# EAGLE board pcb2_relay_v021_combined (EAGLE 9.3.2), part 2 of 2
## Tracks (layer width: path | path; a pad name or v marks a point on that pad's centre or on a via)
+5V  (via drill 0.35)
  Top 0.508: IC1.16 20.95,33.66 21.59,34.29 v21.59,34.81
  Top 0.61: 17.78,26.04 v17.78,15.24 17.78,7.49 18.29,6.99 IC3.10 | 17.78,26.04 17.78,26.85 16.87,27.76 16.87,30.95 17.78,31.86 v17.78,34.92 v17.78,38.1 | IC1.10 17.78,26.04 | v132.08,38.1 v132.08,34.29 132.08,32.48 131.29,31.69 131.29,26.57 131.83,26.04 IC2.10 | v135.26,33.66 IC2.16 | IC3.16 20.45,14.61 20.57,14.73 20.57,15.11 v20.45,15.24
  Top 1.016: IC130.3 C1.+ 22.35,73.66 22.73,73.28 v22.73,72.14 21.21,70.61 21.21,50.16 19.18,48.13 19.18,39.5 v17.78,38.1
  Bottom 0.508: v21.59,34.81 19.29,34.81 C1P.1
  Bottom 0.61: v17.78,15.24 C3P.1 v20.45,15.24 | v17.78,34.92 C1P.1 | v17.78,38.1 v132.08,38.1 | v132.08,34.29 C2P.1 134.62,34.29 v135.26,33.66
  Bottom 1.016: IC130.3 C8.1 22.73,72.09 22.73,72.08 v22.73,72.14
+12V  (via drill 0.35)
  Top 1.016: v24.13,66.42 C15.+ 24.13,63.5 v25.4,63.5 25.4,57.15 24.41,56.16 24.41,50.9 24.44,50.87 K20.1 | K20.1 v26.67,30.48 | v36.83,30.48 K21.1 | v46.99,30.48 v46.98,30.47 K22.1 | v57.15,30.48 K23.1 | v67.31,30.48 K24.1 | v77.47,30.48 v77.46,30.47 K17.1 | v87.63,30.48 K18.1 | v97.79,30.48 K19.1 | v107.95,30.48 K15.1 | v118.11,30.48 K16.1 | v26.67,11.43 K1.1 24.13,11.73 24.13,19.68 22.88,20.93 22.88,29.86 23.48,30.47 K20.1 | v36.83,11.43 K2.1 | v46.99,11.43 K3.1 | v57.15,11.43 K4.1 | v67.31,11.43 v67.3,11.42 K5.1 | v77.47,11.43 K6.1 | v87.63,11.43 v87.62,11.42 K7.1 | v97.79,11.43 K8.1 | v107.95,11.43 K9.1 | v118.11,11.43 K10.1 | v128.27,11.43 K11.1 | v138.43,11.43 v138.42,11.42 K12.1 | v148.59,11.43 v148.58,11.42 K13.1
  Bottom 1.016: IC120.3 17.78,60.96 20.45,63.63 C16.1 | IC130.1 22.86,68.58 24.13,67.31 v24.13,66.42 C16.1 | 35.56,30.48 v26.67,30.48 25.89,29.7 DS20.C | 35.56,30.48 v36.83,30.48 45.72,30.48 | 45.72,30.48 v46.99,30.48 55.88,30.48 | 55.88,30.48 v57.15,30.48 66.04,30.48 | 66.04,30.48 v67.31,30.48 76.2,30.48 | 76.2,30.48 v77.47,30.48 86.36,30.48 | 86.36,30.48 v87.63,30.48 96.52,30.48 | 96.52,30.48 v97.79,30.48 106.68,30.48 | 106.68,30.48 v107.95,30.48 116.84,30.48 | 116.84,30.48 v118.11,30.48 | DS21.C 36.05,29.99 35.56,30.48 | DS22.C 46.21,29.99 45.72,30.48 | DS23.C 56.37,29.99 55.88,30.48 | DS24.C 66.53,29.99 66.04,30.48 | DS17.C 76.69,29.99 76.2,30.48 | DS18.C 86.85,29.99 86.36,30.48 | DS19.C 97.01,29.99 96.52,30.48 | DS15.C 107.17,29.99 106.68,30.48 | DS16.C 117.33,29.99 116.84,30.48 | 35.56,11.43 v26.67,11.43 25.89,10.65 DS1.C | 35.56,11.43 v36.83,11.43 45.72,11.43 | 45.72,11.43 v46.99,11.43 55.88,11.43 | 55.88,11.43 v57.15,11.43 66.04,11.43 | 66.04,11.43 v67.31,11.43 76.2,11.43 | 76.2,11.43 v77.47,11.43 86.36,11.43 | 86.36,11.43 v87.63,11.43 96.52,11.43 | 96.52,11.43 v97.79,11.43 106.68,11.43 | 106.68,11.43 v107.95,11.43 116.84,11.43 | 116.84,11.43 v118.11,11.43 127,11.43 | 127,11.43 v128.27,11.43 137.16,11.43 | 137.16,11.43 v138.43,11.43 147.32,11.43 | 147.32,11.43 v148.59,11.43 | DS13.C 147.81,10.94 147.32,11.43 | DS12.C 137.65,10.94 137.16,11.43 | DS11.C 127.49,10.94 127,11.43 | DS10.C 117.33,10.94 116.84,11.43 | DS9.C 107.17,10.94 106.68,11.43 | DS7.C 86.85,10.94 86.36,11.43 | DS6.C 76.69,10.94 76.2,11.43 | DS5.C 66.53,10.94 66.04,11.43 | DS4.C 56.37,10.94 55.88,11.43 | DS3.C 46.21,10.94 45.72,11.43 | DS2.C 36.05,10.94 35.56,11.43
  Bottom 1.016: DS8.C 97.01,10.94 96.52,11.43 | v25.4,63.5 25.27,63.63 C16.1
+15V  (via drill 0.35)
  Top 0.61: IC13.7 108.2,73.03 v107.44,73.79 | v117.6,73.03 IC15.7 | v111.76,73.66 v111.76,67.31 v111.76,54.99 | v121.92,67.31 v121.92,73.66 | IC12.7 94.61,67.94 v94.74,68.07 | v172.21,70.48 IC21.7 | IC24.7 v172.21,56.52 | v172.09,45.09 IC23.7 | v142.24,60.83 v142.24,54.25 142.98,54.25 143.51,53.72 v143.51,47.12 v143.51,39.37 | v133.86,46.35 IC19.7 | v176.15,71.12 176.15,61.47 176.53,61.09 v176.53,59.69 v176.53,57.15 v176.53,52.32 v176.53,45.97 176.53,43.81 178.44,41.91 v178.44,29.46 | IC17.7 133.73,61.59 v132.97,62.36 | v118.75,52.83 118.87,52.7 IC18.7 | IC16.7 101.73,52.7 v101.09,53.34 | v84.45,52.7 IC14.7 | IC11.7 76.45,67.94 v75.69,68.71 | IC10.7 60.96,67.94 60.71,68.2 v60.71,68.71 | C37.+ 10.31,57.3 13.97,60.96 v13.97,72.39 | IC7.7 177.93,27.3 178.44,27.81 v178.44,27.94 | v183.64,27.3 IC8.7 | v169.04,27.3 IC6.7
  Top 1.016: +15V.TP C35.+ 7.62,46.99 v7.62,48.26 | C18.+ 17.78,48.07 v17.78,48.26 IC120.1 | C37.+ 11.94,54.48 v12.06,54.48
  Bottom 0.61: 176.53,29.46 168.15,29.46 167.64,28.96 C6P.1 168.27,28.07 v169.04,27.3 | 176.53,29.46 v178.44,29.46 184.78,29.46 185.42,28.83 C8P.1 184.41,28.07 v183.64,27.3 | 176.53,29.46 C7P.1 178.31,28.07 v178.44,27.94 | v94.74,68.07 94.1,68.71 C12P.1 92.71,67.44 92.84,67.31 | v107.44,73.79 C13P.1 109.35,73.66 v111.76,73.66 | v117.6,73.03 118.37,73.79 C15P.1 119.51,73.66 v121.92,73.66 | v121.92,67.31 v111.76,67.31 109.18,67.31 108.04,68.45 101.6,68.45 101.47,68.58 99.19,68.58 97.92,67.31 92.84,67.31 | v172.21,70.48 172.98,71.25 C21P.1 176.02,71.25 v176.15,71.12 | v172.21,56.52 172.98,57.28 C24P.1 174.12,57.15 v176.53,57.15 | v172.09,45.09 172.85,45.85 C23P.1 176.41,45.85 v176.53,45.97 183.13,45.97 184.15,46.99 R120.1 | R116.2 169.32,52.32 v176.53,52.32 | v176.53,59.69 165.74,59.69 165.1,59.05 157.86,59.05 157.38,59.54 R102.2 150.65,59.54 149.35,60.83 v142.24,60.83 138.43,60.83 136.9,62.36 C17P.1 v132.97,62.36 | R101.1 v142.24,54.25 142.22,54.23 141.32,54.23 141.29,54.25 140.65,54.25 140.62,54.23 135.64,54.23 134.87,54.99 120.78,54.99 | v133.86,46.35 134.62,47.12 C19P.1 v143.51,47.12 | v118.75,52.83 119.38,53.47 C18P.1 120.78,53.6 120.78,54.99 | v101.09,53.34 101.22,53.47 C16P.1 103,53.6 103,54.99 | v84.45,52.7 85.22,53.47 C14P.1 87.76,53.47 89.28,54.99 103,54.99 | 103,54.99 v111.76,54.99 120.78,54.99 | 77.47,67.31 92.84,67.31 | v75.69,68.71 C11P.1 77.47,67.31 | v60.71,68.71 C10P.1 62.23,67.31 | 77.47,67.31 62.23,67.31 | 62.23,67.31 49.53,67.31 45.72,71.12 21.59,71.12 20.32,72.39 v13.97,72.39 | v143.51,39.37 147.07,39.37 147.32,39.62 R115.1
  Bottom 1.016: +15V.TP C29.1 7.62,47.12 v7.62,48.26 8.93,48.26 9.22,48.55 11.36,48.55 11.65,48.26 v17.78,48.26 | v17.78,48.26 17.78,47.12 C14.1 | v17.78,48.26 19.05,49.53 L7.1 | v12.06,54.48 17.65,54.48 IC120.1
-15V  (via drill 0.35)
  Top 0.305: v7.62,57.15 7.46,57.3 C38.-
  Top 0.508: IC6.4 v163.96,24.77
  Top 0.61: v164.21,23.62 165.48,24.89 v165.48,43.05 165.48,52.96 v165.1,53.34 165.1,58.42 166.37,59.69 v166.37,66.04 v166.37,68.45 | IC21.4 v170.43,67.94 | v170.81,42.55 IC23.4 | v153.67,52.07 IC22.14 | v140.97,53.47 139.7,53.47 v139.7,41.78 | v127,53.98 v127,55.88 v127,59.69 | v131.32,59.05 IC17.4 | v132.72,43.81 IC19.4 | v113.67,50.67 v113.67,55.88 v113.67,69.22 | v99.57,50.16 IC16.4 | v94.49,55.88 v94.49,50.67 | v83.19,50.16 IC14.4 | v78.74,50.8 v78.74,55.88 v78.74,60.96 | v89.53,65.41 IC12.4 | v85.6,65.91 v85.6,55.88 | v74.3,65.41 IC11.4 | v59.05,65.41 IC10.4 | v116.2,70.48 IC15.4 | v106.05,70.48 IC13.4 | v57.15,64.26 v57.15,60.96 | v72.39,60.96 v72.39,64.26 | IC20.14 v153.67,66.04 | IC24.4 v170.69,53.98 | v182.12,24.77 IC8.4 | v172.85,24.77 IC7.4 | v117.22,50.16 IC18.4
  Top 1.016: -15V.TP 5.08,68.58 C36.- v8.89,68.58 8.89,66.04 7.46,64.61 C38.-
  Bottom 0.305: L5.1 8.89,55.88 v7.62,57.15
  Bottom 0.508: C6N.2 163.45,25.27 v163.96,24.77
  Bottom 0.61: C6N.2 162.56,24.13 163.07,23.62 v164.21,23.62 171.45,23.62 | 171.45,23.62 179.83,23.62 180.34,24.13 C8N.2 181.61,25.27 v182.12,24.77 | 171.45,23.62 C7N.2 172.34,25.27 v172.85,24.77 | v170.43,67.94 169.41,67.94 C21N.2 v166.37,68.45 | v170.81,42.55 170.31,43.05 C23N.2 v165.48,43.05 | 144.78,53.48 143.69,53.48 143.68,53.47 v140.97,53.47 127.51,53.47 v127,53.98 | 144.78,53.48 147.18,53.48 148.59,52.07 v153.67,52.07 156.21,52.07 157.48,53.34 v165.1,53.34 R122.1 168.89,54.46 C24N.2 170.18,54.48 v170.69,53.98 | R108.2 144.78,53.48 | v127,59.69 129.41,59.69 C17N.2 130.81,59.56 v131.32,59.05 | v132.72,43.81 132.21,44.32 C19N.2 130.81,42.55 131.57,41.78 v139.7,41.78 142.22,41.78 R110.2 | v113.67,50.67 C18N.2 116.72,50.67 v117.22,50.16 | v127,55.88 v113.67,55.88 v94.49,55.88 v85.6,55.88 v78.74,55.88 | v99.57,50.16 99.06,50.67 C16N.2 v94.49,50.67 | v83.19,50.16 82.68,50.67 C14N.2 78.87,50.67 v78.74,50.8 | v89.53,65.41 89.03,65.91 C12N.2 v85.6,65.91 | v74.3,65.41 73.79,65.91 C11N.2 v72.39,64.26 | C10N.2 58.55,65.91 v59.05,65.41 | v116.2,70.48 115.7,70.99 C15N.2 114.3,69.85 v113.67,69.22 104.14,69.22 C13N.2 105.54,70.99 v106.05,70.48 | C10N.2 48.52,65.91 44.58,69.85 11.37,69.85 11.28,69.94 9.23,69.94 8.89,69.6 v8.89,68.58 | v57.15,60.96 v72.39,60.96 v78.74,60.96 | C10N.2 v57.15,64.26 | v153.67,66.04 v166.37,66.04
  Bottom 0.813: v8.89,68.58 C30.2
  Bottom 1.016: C30.2 5.08,68.58 -15V.TP
A  (via drill 0.35)
  Top 0.305: K20.6 32.41,26.04 v33.02,26.04 33.63,26.04 K21.3 | v63.5,26.04 64.11,26.04 K24.3 | K23.3 53.95,26.04 v53.34,26.04 | K22.3 43.8,26.04 v43.18,26.04 43.18,40.64 39.37,44.45 C22.1 39.37,49.53 40.64,50.8 40.64,58.42 v39.37,59.69
  Bottom 0.305: v33.02,26.04 v43.18,26.04 v53.34,26.04 v63.5,26.04 | L4.2 v39.37,59.69
AD_LVL  (via drill 0.35)
  Top 0.305: v154.94,25.4 v154.94,33.02
  Bottom 0.305: R1.2 v154.94,33.02 R193.1 | v154.94,25.4 143.51,25.4 142.24,26.67 6.02,26.67 4.75,25.4 CON2.2
E12  (via drill 0.35)
  Top 0.305: IC9.3 52.2,56.52 v52.83,57.15 | K20.5 28.14,26.17 28.14,33.59 26.67,35.06 26.67,54.61 v29.21,57.15
  Bottom 0.305: R50.2 59.69,56.52 59.05,57.15 53.34,57.15 v52.83,57.15 48.97,57.15 47.45,58.67 46.35,58.67 44.83,57.15 v29.21,57.15
E13  (via drill 0.35)
  Top 0.305: C23.+ 54.61,50.8 v55.88,52.07 | K20.4 26.68,22.87 27.69,23.88 27.69,33.4 25.4,35.69 v25.4,51.31
  Bottom 0.305: R53.2 59.84,52.07 v55.88,52.07 45.47,52.07 44.7,51.31 v25.4,51.31
E15  (via drill 0.35)
  Top 0.305: K20.3 26.11,25.07 v26.16,25.02 | v50.16,25.02 51.71,25.02 K22.6 | v60.2,25.02 60.25,25.07 K23.6 | K24.6 72.03,25.02 v70.48,25.02 69.09,26.42 69.09,31.38 67.82,32.65 v67.82,59.69 67.82,60.2 68.58,60.96 68.58,64.77 67.31,66.04 v67.31,68.96 66.04,70.23 v66.04,73.91 | K21.4 33.52,22.87 33.02,23.37 v33.02,25.02 | IC17.3 126.36,60.33 v125.73,59.69
  Bottom 0.305: v26.16,25.02 v33.02,25.02 v50.16,25.02 v60.2,25.02 v70.48,25.02 | E15.TP 56.44,74.93 57.45,73.91 v66.04,73.91 | v67.31,68.96 R54.2 | v125.73,59.69 v67.82,59.69
E16  (via drill 0.35)
  Top 0.305: v22.86,5.08 22.86,4.32 23.37,3.81 23.38,3.82 K1.4 24.13,3.51 v24.13,1.91 | v115.82,1.91 115.82,3.76 K10.4 | K9.4 105.72,1.96 v105.66,1.91 | K8.4 95.56,1.96 v95.5,1.91 | K7.4 85.47,3.75 v85.47,1.91 | v75.18,1.91 75.24,1.96 K6.4 74.03,5.03 74.03,31.2 75.24,32.4 75.24,66.35 | K5.4 65.08,1.96 v65.02,1.91 | K4.4 54.92,1.96 v54.86,1.91 | K3.4 44.76,1.96 v44.7,1.91 | K2.4 34.6,1.96 v34.54,1.91 | 75.24,66.35 75.56,66.67 IC11.6 | 75.24,66.35 75.24,67.64 74.93,67.94 v74.93,74.93
  Bottom 0.305: RG1.1 20.17,5.08 v22.86,5.08 | v24.13,1.91 v34.54,1.91 v44.7,1.91 v54.86,1.91 v65.02,1.91 v75.18,1.91 v85.47,1.91 v95.5,1.91 v105.66,1.91 v115.82,1.91 | v74.93,74.93 72.29,74.93 R61.2 70.7,76.52 53.02,76.52 E16.TP
E17  (via drill 0.35)
  Top 0.305: v139.7,6.6 139.7,12.7 138.43,13.97 138.43,19.05 139.7,20.32 139.7,26.67 138.43,27.94 COQ1.2 v138.43,64.77 | v99.06,64.77 v99.06,72.39
  Bottom 0.305: RG11.2 137.16,6.35 137.41,6.6 v139.7,6.6 | v138.43,64.77 v99.06,64.77 | E17.TP 63.99,76.97 72.38,76.97 73.66,75.69 86.74,75.69 87.76,74.68 87.63,74.55 R213.1 88.04,73.41 96.01,73.41 96.9,72.52 98.93,72.52 v99.06,72.39 | COQ4.2 156.46,30.73 151.38,30.73 COQ3.1 144.78,30.48 | COQ1.2 144.78,30.48 | COQ2.2 144.78,30.48
E18  (via drill 0.35)
  Top 0.305: K11.4 126.04,3.5 v127,2.54 | v156.21,2.54 v156.21,16.51 156.21,20.32 154.94,21.59 v154.94,22.86 154.94,24.51 154.31,25.14 154.31,42.54 v153.67,43.18 | K13.4 146.05,3.51 v146.05,2.54 | K12.4 136.2,2.61 v136.27,2.54 | IC12.6 90.3,66.67 | 90.3,66.67 90.3,64.77 90.17,64.64 v90.17,60.96 | 90.3,66.67 v90.3,74.93 90.3,77.19 v90.16,77.33 | v142.24,43.18 C47.+ 142.09,49.53 v140.97,49.53 | v123.19,50.04 123.19,59.56 v121.79,60.96
  Bottom 0.305: v127,2.54 v136.27,2.54 v146.05,2.54 v156.21,2.54 | v154.94,22.86 153.67,24.13 R81.1 | E18.TP 82.55,78.74 R62.2 R62.1 90.02,77.47 v90.16,77.33 | R63.2 v90.3,74.93 | v153.67,43.18 v142.24,43.18 | v140.97,49.53 130.81,49.53 130.3,50.04 v123.19,50.04 | v90.17,60.96 v121.79,60.96 121.79,62.2 R84.2 | v156.21,16.51 ROQ4.1
E19  (via drill 0.35)
  Top 0.305: K1.5 31.75,3.81 v33.02,2.54 | v43.18,2.54 41.9,3.82 K2.5 | v53.34,2.54 52.06,3.82 K3.5 | v63.5,2.54 63.2,2.54 K4.5 | v73.66,2.54 73.36,2.54 K5.5 | v83.82,2.54 83.52,2.54 K6.5 | v93.98,2.54 93.68,2.54 K7.5 | v104.14,2.54 102.86,3.82 K8.5 | v114.3,2.54 114,2.54 K9.5 | v124.46,2.54 123.18,3.82 K10.5 | v88.9,2.54 88.9,13.34 87.63,14.61 87.63,20.19 88.9,21.46 88.9,31.88 87.76,33.02 v87.76,43.05 87.76,48.39 88.9,49.53 v88.9,60.96 | v106.68,61.59 v106.68,66.04 106.68,71.75 | 106.68,71.75 106.68,74.93 v104.78,76.83 | 106.68,71.75 IC13.6
  Bottom 0.305: RH1.1 v33.02,2.54 v43.18,2.54 v53.34,2.54 v63.5,2.54 v73.66,2.54 v83.82,2.54 v88.9,2.54 v93.98,2.54 v104.14,2.54 v114.3,2.54 v124.46,2.54 | R70.2 90.14,43.05 v87.76,43.05 80.03,43.05 R69.2 R67.2 | v106.68,66.04 R64.2 | E19.TP 94.61,76.83 v104.78,76.83 | v88.9,60.96 89.28,60.96 89.91,61.59 90.43,61.59 90.61,61.42 106.5,61.42 v106.68,61.59
E20  (via drill 0.35)
  Top 0.305: v129.54,12.7 v129.54,3.81 | CPR1.2 158.75,15.62 159.38,16.25 159.38,16.77 158.75,17.4 158.75,53.34 160.02,54.61 v160.02,64.77 | v110.49,66.04 111,66.55 111,75.69 v110.49,76.2
  Bottom 0.305: v129.54,3.81 RH11.2 | v129.54,12.7 CPR1.2 165.1,12.7 | v110.49,76.2 R214.1 106.68,76.2 E20.TP | v110.49,66.04 152.78,66.04 153.41,65.41 159.38,65.41 v160.02,64.77 | CPR4.2 176.53,12.7 CPR3.1 165.1,12.7 | CPR2.2 165.1,12.7
E21  (via drill 0.35)
  Top 0.305: K11.5 133.04,1.96 v133.1,1.91 | v154.94,1.91 154.94,3.81 | 154.94,3.81 v154.94,6.35 | K13.5 154.93,3.82 154.94,3.81 | K12.5 | K12.5 143.2,1.98 v143.13,1.91 | K12.5 141.22,3.81 140.33,4.7 140.33,13.71 139.07,14.98 139.07,19.04 140.16,20.13 140.16,37.64 v139.7,38.1 | E21.TP 116.84,77.47 v116.84,76.2 116.84,71.75 | 109.6,53.21 v109.6,43.05 v109.6,38.88 | 109.6,53.21 v109.6,64.14 | v116.84,64.14 116.84,71.75 | IC15.6 116.84,71.75 | v108.58,53.21 109.6,53.21
  Bottom 0.305: v133.1,1.91 v143.13,1.91 v154.94,1.91 | R77.2 R78.2 109.58,43.03 v109.6,43.05 | v116.84,76.2 123.19,76.2 R59.2 R59.1 128.27,78.74 139.7,78.74 CON1.4 | R79.2 106.96,53.21 v108.58,53.21 | v109.6,64.14 v116.84,64.14 | v109.6,38.88 109.78,38.71 131.8,38.71 131.82,38.73 139.07,38.73 v139.7,38.1 | v154.94,6.35 155.57,6.99 163.45,6.99 163.83,7.37 165.99,7.37 167,6.35 RPR4.1
E22  (via drill 0.35)
  Top 0.305: v160.02,74.93 E22.TP | v93.85,58.55 93.6,58.29 93.59,58.29 92.33,57.03 v92.33,43.05 | v124.46,58.55 124.46,63.37 127,65.91 v127,72.39 | v146.05,72.77 CON1.7
  Bottom 0.305: CON1.7 v160.02,74.93 | R71.1 92.35,43.03 v92.33,43.05 | v93.85,58.55 v124.46,58.55 | v127,72.39 127.38,72.77 v146.05,72.77
E23  (via drill 0.35)
  Top 0.305: v110.49,52.07 v110.49,63.5 | v136.53,63.5 v136.53,79.38
  Bottom 0.305: E23.TP 166.34,80.03 148.62,80.03 147.96,79.38 147.83,79.38 147.32,79.38 146.18,79.38 | R80.1 v110.49,52.07 | v110.49,63.5 v136.53,63.5 | v136.53,79.38 146.18,79.38 | CON1.8 146.05,79.25 146.18,79.38
E24
  Bottom 0.305: R81.2 156.36,25.4 | 156.36,25.4 R82.1 | R182.2 158.6,25.4 156.36,25.4
E25  (via drill 0.35)
  Top 0.305: K15.4 105.72,20.7 v105.92,20.5 | v118.62,20.5 118.62,28.83 118.92,29.13 118.92,31.56 117.65,32.83 117.65,40.34 v116.08,41.91
  Bottom 0.305: v105.92,20.5 v118.62,20.5 | R88.2 v116.08,41.91
E26  (via drill 0.35)
  Top 0.305: C42.+ 120.65,38.1 118.11,35.56 118.11,33.02 119.38,31.75 v119.38,22.86
  Bottom 0.305: R90.1 80.16,22.71 81.28,21.59 119.53,21.59 R94.2 v119.38,22.86
E28  (via drill 0.35)
  Top 0.305: K17.3 76.66,25.07 v76.71,25.02 | K18.6 93.93,25.07 v93.98,25.02 94.03,25.07 K19.3 | K16.3 115.83,25.02 v114.3,25.02 v114.3,48.26 | IC19.3 129.03,45.09 v128.27,45.85 127,47.12 E28.TP
  Bottom 0.305: v76.71,25.02 v93.98,25.02 v114.3,25.02 | v114.3,48.26 E28.TP | v128.27,45.85 R123.2
E29  (via drill 0.35)
  Top 0.305: E29.TP C46.- 180.5,73.5 v180.34,73.66
  Bottom 0.305: R105.1 184,69.85 E29.TP | CON1.3 142.24,73.66 153.41,73.66 154.04,73.03 165.1,73.03 165.67,72.45 173.8,72.45 175,73.66 v180.34,73.66
E31  (via drill 0.35)
  Top 0.305: IC24.6 v175.64,55.24 | v135.76,65.41 v135.76,77.47 | v178.09,51.18 178.09,55.88 | 178.09,55.88 178.09,61.94 C51.2 v177.8,64.77 | v179.07,55.88 178.09,55.88
  Bottom 0.305: v175.64,55.24 178.44,55.24 v179.07,55.88 180.34,57.15 E31.TP | R124.2 177.86,50.95 v178.09,51.18 | v135.76,65.41 135.94,65.58 152.59,65.58 153.27,64.9 156.84,64.9 157.61,64.14 161.04,64.14 161.67,64.77 v177.8,64.77 | v135.76,77.47 CON1.2
GND  (via drill 0.35)
  Top 0.305: IC1.13 17.93,29.84 v17.91,29.82 | IC3.13 v21.21,10.79 | IC2.13 134.88,29.84 v135.51,29.21 | R75.1 v97.79,47.15 | IC24.3 v170.69,55.24
  Bottom 0.305: C21N.1 v170.56,71.25 | R55.1 v70.48,65.79 | C13N.1 102.36,73.79 v102.23,73.91
  Bottom 0.61: R109.1 v144.78,40.39
  pour Top (isolate 0.406): 0,82.55 189.23,82.55 189.23,0 0,0
  pour Bottom (isolate 0.305): 0,82.55 189.23,82.55 189.23,0 0,0
IC9+15V  (via drill 0.35)
  Top 0.305: v33.02,49.53 C9P1.+ | v58.42,49.42 58.42,57.67 v58.31,57.78 IC9.7
  Bottom 0.305: L7.2 v33.02,49.53 58.31,49.53 v58.42,49.42 | v58.31,57.78 57.54,58.55 C9P.1
IC9-15V  (via drill 0.35)
  Top 0.305: v33.02,55.88 C9N1.- 34.45,54.77 v35.56,55.88 | v48.9,55.24 IC9.4
  Bottom 0.305: L5.2 v33.02,55.88 | v35.56,55.88 48.26,55.88 48.39,55.75 | 48.39,55.75 v48.9,55.24 | C9N.2 48.39,55.75
IC10P5  (via drill 0.35)
  Top 0.305: IC10.5 63.63,65.41 64.01,65.02 v64.01,63.48
  Bottom 0.305: v64.01,63.48 52.09,63.48 C24.2
IC11P5  (via drill 0.35)
  Top 0.305: v75.87,63.5 75.87,65.08 76.2,65.41 IC11.5
  Bottom 0.305: C25.2 v75.87,63.5
IC12P5
  Top 0.305: IC12.5 95.63,65.41 96.14,64.9 C26.2
IC13P5  (via drill 0.35)
  Top 0.305: IC13.5 107.82,70.48 107.57,70.23 v107.57,67.57
  Bottom 0.305: v107.57,67.57 100.84,67.57 C27.2
IC15P5  (via drill 0.35)
  Top 0.305: IC15.5 v121.03,70.48
  Bottom 0.305: v121.03,70.48 121.67,69.85 129.54,69.85 C28.2
IN
  Top 0.305: C211.1 INPUT.TP
  Bottom 0.305: C210.1 C211.1
IREF  (via drill 0.35)
  Top 0.305: C49.+ 162.41,44.6 v162.56,44.45 | IC23.6 v171.45,43.81 171.45,48.11 R117.2 | v180.34,44.56 180.34,50.8 180.19,50.95 C50.- 179.07,54.99 180.14,56.05 180.14,62.67 179.07,63.74 179.07,74.93 E32.TP
  Bottom 0.305: CON1.1 139.7,76.2 172.72,76.2 E32.TP | v162.56,44.45 170.81,44.45 v171.45,43.81 171.83,43.81 172.58,44.56 v180.34,44.56
N$1  (via drill 0.35)
  Top 0.305: IC6.3 161.04,26.04 v160.02,27.05
  Bottom 0.305: v160.02,27.05 158.98,28.09 R182.1
N$2  (via drill 0.35)
  Top 0.305: v177.8,22.84 177.8,25.15 178.69,26.04 IC8.3
  Bottom 0.305: R190.2 v177.8,22.84
N$3  (via drill 0.35)
  Top 0.305: K19.4 94.3,24.13 v93.98,24.13
  Bottom 0.305: R93.1 R92.2 99.21,24.13 v93.98,24.13
N$4  (via drill 0.35)
  Top 0.305: v93.98,22.86 K18.5
  Bottom 0.305: R91.2 v93.98,22.86 R92.1
N$5  (via drill 0.35)
  Top 0.305: K17.4 v78.73,22.87 v78.74,22.86
  Bottom 0.305: v78.74,22.86 R90.2 78.59,24.13 86.36,24.13 87.48,23.01 R91.1
N$6  (via drill 0.35)
  Top 0.305: K16.4 v114.31,22.87 v114.3,22.86
  Bottom 0.305: v114.3,22.86 R94.1
N$7  (via drill 0.35)
  Top 0.305: QS19.1 99.23,34.46 v99.06,34.29
  Bottom 0.305: v99.06,34.29 100.18,35.41 RS19.1
N$8  (via drill 0.35)
  Top 0.508: v101.09,29.34 101.6,29.84 101.6,30.48 | QS19.3 101.6,30.48 | K19.8 101.61,30.47 101.6,30.48
  Bottom 0.508: DS19.A 101.11,29.32 v101.09,29.34
N$10  (via drill 0.35)
  Top 0.305: IC6.2 161.04,27.3 160.66,27.69 160.66,33.15 v161.8,34.29
  Bottom 0.305: R183.1 160.17,34.29 v161.8,34.29 R184.2
N$11  (via drill 0.35)
  Top 0.305: C73.+ 166.56,33.02 v166.37,33.02 166.37,26.16 166.5,26.04 IC6.6
  Bottom 0.305: v166.37,33.02 166.52,33.17 R184.1
N$12  (via drill 0.35)
  Top 0.305: v63.5,70.99 63.68,70.82 63.68,69.39 63.5,69.22 IC10.8
  Bottom 0.305: C24.1 63.38,71.12 v63.5,70.99
N$13
  Bottom 0.305: R192.1 151.54,36.98 R193.2
N$14  (via drill 0.35)
  Top 0.305: v169.93,21.97 169.93,27.3 | 169.93,27.3 v169.93,30.35 | IC7.2 169.93,27.3
  Bottom 0.305: R187.2 170.16,21.74 v169.93,21.97 | R186.1 R185.1 169.93,31.34 v169.93,30.35
N$15  (via drill 0.35)
  Top 0.305: v171.45,17.78 173.15,17.78 D23.1
  Bottom 0.305: R187.1 v171.45,17.78
N$16
  Top 0.305: D23.2 173.99,25.53 174.5,26.04 | 174.5,26.04 IC7.6 | 174.5,26.04 174.5,30.61 175.21,31.32 D22.1
N$17  (via drill 0.35)
  Top 0.305: v127,62.23 127.64,61.59 IC17.2 131.44,61.59 132.33,60.71 v132.33,57.32
  Bottom 0.305: v127,62.23 R84.1 | v132.33,57.32 131.72,57.32 R85.2
N$18  (via drill 0.35)
  Top 0.305: R188.1 180.23,34.56 180.34,34.67 v181.61,34.67 | v175.26,34.42 176.23,34.42 D22.2
  Bottom 0.305: R186.2 174.01,34.42 v175.26,34.42 181.36,34.42 v181.61,34.67
N$19  (via drill 0.35)
  Top 0.305: R188.2 182.37,31.6 | 182.37,31.6 R189.1 | C74.- 182.88,17.93 v182.88,20.32 182.88,27.3 | 182.88,27.3 182.88,29.72 182.37,30.23 182.37,31.6 | IC8.2 182.88,27.3
  Bottom 0.305: R191.1 v182.88,20.32
N$20  (via drill 0.35)
  Top 0.305: v187.96,35.56 187.96,26.04 | 187.96,26.04 v187.96,20.32 187.96,18.16 187.58,17.78 C74.+ | IC8.6 187.96,26.04
  Bottom 0.305: R192.3 R192.2 149.35,35.56 v187.96,35.56 | R191.2 v187.96,20.32
N$22  (via drill 0.35)
  Top 0.305: IC17.6 136.53,60.33 137.16,59.69 137.16,56.64 v137.03,56.52 | C41.- 131.57,52.07 132.33,52.83 v132.33,56.52
  Bottom 0.305: v137.03,56.52 R85.1 v132.33,56.52
N$23  (via drill 0.35)
  Top 0.305: v172.34,33.27 172.53,33.47 C73.- | v182.75,33.27 183.92,34.44 R189.2
  Bottom 0.305: R185.2 171.35,33.27 v172.34,33.27 v182.75,33.27
N$24  (via drill 0.35)
  Top 0.305: IC18.3 v117.22,51.44 | C41.+ v124.46,52.07
  Bottom 0.305: v117.22,51.44 118.75,51.44 119.38,52.07 v124.46,52.07 R86.2
N$26  (via drill 0.35)
  Top 0.305: IC10.6 63.75,66.67 64.14,67.06 v64.14,75.06
  Bottom 0.305: R60.1 R56.2 64.11,75.08 v64.14,75.06
N$27  (via drill 0.35)
  Top 0.305: IC11.2 70.99,67.94 70.48,68.45 v70.48,75.31
  Bottom 0.305: R60.2 59.52,73.34 65.34,73.34 65.41,73.28 66.42,73.28 68.45,75.31 R61.1 v70.48,75.31
N$28  (via drill 0.35)
  Top 0.305: IC18.2 117.6,52.7 117.98,52.32 v117.98,46.99
  Bottom 0.305: R89.2 116.71,46.97 | 116.71,46.97 C75.2 117.37,43.79 R88.1 | v117.98,46.99 117.96,46.97 116.71,46.97
N$29  (via drill 0.35)
  Top 0.305: C42.- 120.84,46.99 v122.17,46.99 122.56,47.37 122.56,51.05 122.17,51.44 IC18.6
  Bottom 0.305: C75.1 119.51,46.97 R89.1 v122.17,46.99
N$30  (via drill 0.35)
  Top 0.305: v22.86,6.35 23.19,6.02 K1.3
  Bottom 0.305: RG1.2 v22.86,6.35 RG2.1
N$31  (via drill 0.35)
  Top 0.305: IC11.8 79.25,69.22 79.5,69.47 v79.5,70.36
  Bottom 0.305: C25.1 78.87,71.12 79.5,70.48 v79.5,70.36
N$32  (via drill 0.35)
  Top 0.305: IC12.2 89.15,67.94 89.41,68.2 v89.41,70.87
  Bottom 0.305: v89.41,70.87 89.31,70.97 R213.2
N$33  (via drill 0.35)
  Top 0.305: v48.9,50.8 C23.- 50.65,51.91 53.34,54.61 53.34,55.88 53.98,56.52 IC9.6
  Bottom 0.305: v48.9,50.8 47.14,50.8 R52.2
N$34  (via drill 0.35)
  Top 0.305: IC9.2 47.24,57.78 v46.99,58.04 | v45.59,53.47 v45.59,57.02
  Bottom 0.305: v46.99,58.04 R51.2 45.62,57 v45.59,57.02 | R52.1 45.62,53.49 v45.59,53.47
N$35
  Top 0.305: IC12.8 95.63,69.22 96.14,69.72 C26.1
N$36  (via drill 0.35)
  Top 0.305: v129.16,46.35 IC19.2 132.72,46.35 133.35,46.99 v133.35,52.07
  Bottom 0.305: R95.1 125.73,45.59 126.62,46.48 128.53,46.48 128.66,46.35 v129.16,46.35 | v133.35,52.07 R96.2
N$37  (via drill 0.35)
  Top 0.305: IC19.6 137.54,45.09 137.92,45.47 137.92,51.95 v137.8,52.07 137.8,63.24 136.98,64.06 136.98,65.61 137.41,66.04 C43.+
  Bottom 0.305: v137.8,52.07 R96.1
N$38  (via drill 0.35)
  Top 0.305: IC10.3 59.05,66.67 59.69,66.04 v64.77,66.04 v64.77,68.96
  Bottom 0.305: v64.77,66.04 65.63,66.04 R55.2 | v64.77,68.96 R54.1
N$39  (via drill 0.35)
  Top 0.305: v85.07,66.53 85.22,66.67 IC12.3
  Bottom 0.305: R83.2 84.43,65.89 v85.07,66.53
N$40  (via drill 0.35)
  Top 0.305: IC13.2 v101.6,73.03 101.6,67.31 v102.87,66.04 103.5,65.41 v103.5,62.05 | R66.2 81.89,62.38 v81.92,62.36 83.8,62.36 R65.1
  Bottom 0.305: R64.1 v102.87,66.04 | v101.6,73.03 101.47,73.15 97.18,73.15 R63.1 | v81.92,62.36 88.38,62.36 88.89,62.86 93.85,62.86 94.66,62.05 v103.5,62.05
N$41  (via drill 0.35)
  Top 0.305: IC13.8 108.2,74.3 v107.57,74.93
  Bottom 0.305: v107.57,74.93 C27.1
N$42  (via drill 0.35)
  Top 0.305: IC14.6 88.01,51.44 88.27,51.69 88.27,57.15 88.27,57.63 88.27,57.78 v87.63,58.42 R72.2 | R65.2 v83.82,58.42
  Bottom 0.305: v83.82,58.42 v87.63,58.42
N$43  (via drill 0.35)
  Top 0.305: IC14.3 79.54,51.44 v79.53,51.45
  Bottom 0.305: v79.53,51.45 77.01,51.45 R68.2 R67.1
N$44
  Bottom 0.305: R71.2 R70.1 87.78,45.87 Q5.G
N$45  (via drill 0.35)
  Top 0.305: 83.82,52.7 83.82,54.61 82.55,55.88 v82.55,60.96 | 83.82,52.7 Q5.D | R72.1 v87.63,60.96 | v92.71,62.23 91.59,62.23 R73.2 | IC14.2 83.82,52.7
  Bottom 0.305: Q5.D 82.4,45.87 R69.1 | v92.71,62.23 88.9,62.23 v87.63,60.96 v82.55,60.96
N$46  (via drill 0.35)
  Top 0.305: IC16.3 97.71,51.46 v95.27,51.46 95.25,51.44 95.25,49.53 95.89,48.9 v95.89,45.85
  Bottom 0.305: R77.1 95.91,45.87 v95.89,45.85 | v95.27,51.46 93.52,51.46 R76.2
N$47  (via drill 0.35)
  Top 0.305: Q6.G 108.58,45.09 v108.58,50.65
  Bottom 0.305: R79.1 v108.58,50.65 R80.2
N$48  (via drill 0.35)
  Top 0.305: R74.1 R75.2 98.91,43.03 100.33,44.45 v100.33,45.72 100.33,52.07 99.69,52.7 IC16.2
  Bottom 0.305: Q6.D 103.99,45.87 R78.1 100.48,45.87 v100.33,45.72
N$49  (via drill 0.35)
  Top 0.305: R66.1 v80.26,57.66 | v93.85,57.66 93.85,46 R74.2 | v104.78,57.66 104.78,51.82 104.39,51.44 IC16.6
  Bottom 0.305: v80.26,57.66 v93.85,57.66 v104.78,57.66
N$51
  Top 0.305: C28.1 123.19,73.79 122.68,74.3 IC15.8
N$52  (via drill 0.35)
  Top 0.305: v115.57,76.2 116.08,75.69 116.08,73.53 115.57,73.03 IC15.2
  Bottom 0.305: R214.2 v115.57,76.2
N$53  (via drill 0.35)
  Top 0.305: v80.01,73.66 80.01,76.2 R62.3
  Bottom 0.305: R57.2 80.16,73.81 v80.01,73.66
N$54  (via drill 0.35)
  Top 0.305: v85.09,74.93 v85.09,80.01
  Bottom 0.305: R58.2 v85.09,74.93 | v85.09,80.01 91.16,80.01 91.18,80.03 119.36,80.03 R59.3
N$55  (via drill 0.35)
  Top 0.305: v33.02,6.35 33.35,6.02 K2.3
  Bottom 0.305: RG2.2 v33.02,6.35 RG3.1
N$56  (via drill 0.35)
  Top 0.305: v60.07,72.26 60.07,69.47 58.55,67.94 IC10.2
  Bottom 0.305: R58.1 R57.1 81.13,71.12 79.88,71.12 78.77,72.24 R56.1 62.2,72.26 v60.07,72.26
N$57  (via drill 0.35)
  Top 0.305: C43.- 142.24,64.92 v142.24,63.5
  Bottom 0.305: v142.24,63.5 R97.2
N$58  (via drill 0.35)
  Top 0.305: IC20.3 v148.59,63.5
  Bottom 0.305: v148.59,63.5 R97.1
N$59  (via drill 0.35)
  Top 0.305: v139.7,59.69 v139.7,61.62 | v148.59,61.62 148.59,61.34 148.21,60.96 IC20.5
  Bottom 0.305: R100.1 v139.7,59.69 | v139.7,61.62 v148.59,61.62
N$60  (via drill 0.35)
  Top 0.305: v149.86,64.77 IC20.2
  Bottom 0.305: R106.1 150.98,63.65 v149.86,64.77
N$61  (via drill 0.35)
  Top 0.305: C45.- 162.59,60.8 v162.56,60.83
  Bottom 0.305: v162.56,60.83 163.81,60.83 R106.2
N$62  (via drill 0.35)
  Top 0.305: v145.91,58.42 145.91,62.1 | 145.91,62.1 145.91,65.64 146.18,65.91 147.03,65.91 IC20.1 | IC20.4 146.03,62.23 145.91,62.1
  Bottom 0.305: R108.1 145.75,58.57 v145.91,58.42 146.06,58.57 R107.2
N$63  (via drill 0.35)
  Top 0.305: v43.18,6.35 44.43,6.35 K3.3
  Bottom 0.305: RG3.2 v43.18,6.35 RG4.1
N$64  (via drill 0.35)
  Top 0.305: IC20.8 154.78,58.42 v154.94,58.26
  Bottom 0.305: v154.94,58.26 R98.1
N$65
  Top 0.305: R99.1 157.63,60.96 IC20.10
N$66  (via drill 0.35)
  Top 0.305: IC20.6 v148.59,59.69
  Bottom 0.305: R101.2 142.24,59.18 142.75,59.69 v148.59,59.69
N$67  (via drill 0.35)
  Top 0.305: v153.67,63.02 153.19,63.5 IC20.12 | v161.67,62.36 161.67,70.58 C44.+
  Bottom 0.305: v153.67,63.02 154.3,63.02 R102.1 161.65,62.38 v161.67,62.36
N$68  (via drill 0.35)
  Top 0.305: v163.83,66.96 C45.+ | IC21.6 v172.21,69.22 171.45,69.98 v171.45,73.66
  Bottom 0.305: D8.2 146.48,69.85 163.83,69.85 | 163.83,69.85 171.58,69.85 v172.21,69.22 | 163.83,69.85 D11.1 v163.83,66.96 | R104.1 175.41,75.08 173.99,73.66 R103.2 v171.45,73.66
N$69  (via drill 0.35)
  Top 0.305: IC21.2 167,70.48 166.37,71.12 | 166.37,71.12 C44.- | 166.37,71.12 v166.37,73.66 | v154.31,73.66 v154.31,71.55
  Bottom 0.305: D6.1 v154.31,71.55 D9.2 | R103.1 v166.37,73.66 v154.31,73.66
N$70
  Bottom 0.305: D9.1 D10.2
N$71  (via drill 0.35)
  Top 0.305: v53.34,6.35 54.59,6.35 K4.3
  Bottom 0.305: RG4.2 v53.34,6.35 RG5.1
N$72  (via drill 0.35)
  Top 0.305: v63.5,6.35 64.75,6.35 K5.3
  Bottom 0.305: RG5.2 v63.5,6.35 RG6.1
N$73  (via drill 0.35)
  Top 0.305: K6.3 75.24,6.67 v74.93,6.99
  Bottom 0.305: RG6.2 70.64,6.99 v74.93,6.99 76.68,6.99 RG7.1
N$74  (via drill 0.35)
  Top 0.305: v83.82,6.35 85.07,6.35 K7.3
  Bottom 0.305: RG7.2 v83.82,6.35 RG8.1
N$75  (via drill 0.35)
  Top 0.305: v93.98,6.35 95.23,6.35 K8.3
  Bottom 0.305: RG8.2 v93.98,6.35 RG9.1
N$76  (via drill 0.35)
  Top 0.305: v104.14,6.35 105.39,6.35 K9.3
  Bottom 0.305: RG9.2 v104.14,6.35 RG10.1
N$77  (via drill 0.35)
  Top 0.305: v114.3,6.35 115.55,6.35 K10.3
  Bottom 0.305: RG10.2 v114.3,6.35 RG11.1
N$78  (via drill 0.35)
  Top 0.305: v27.94,3.81 27.94,5.33 28.57,5.97 31.39,5.97 K1.6
  Bottom 0.305: v27.94,3.81 RH2.1 19.05,3.81 18.9,3.66 RH1.2
N$79  (via drill 0.35)
  Top 0.305: v43.18,5.08 42.24,6.02 K2.6
  Bottom 0.305: v43.18,5.08 41.91,3.81 RH3.1 38.25,5.08 30.63,5.08 RH2.2
N$80  (via drill 0.35)
  Top 0.305: v53.34,5.08 52.7,5.08 K3.6 | v38.1,3.81 v38.1,7.62 | v48.26,7.62 v48.26,5.08
  Bottom 0.305: RH4.1 48.11,5.08 v48.26,5.08 v53.34,5.08 | RH3.2 v38.1,3.81 | v38.1,7.62 v48.26,7.62
N$81  (via drill 0.35)
  Top 0.305: v63.5,5.08 62.86,5.08 K4.6
  Bottom 0.305: RH4.2 RH5.1 58.27,5.08 v63.5,5.08
N$82  (via drill 0.35)
  Top 0.305: v73.15,5.08 73.02,5.08 K5.6
  Bottom 0.305: RH5.2 RH6.1 68.43,5.08 v73.15,5.08
N$83  (via drill 0.35)
  Top 0.305: v83.82,5.08 83.18,5.08 K6.6
  Bottom 0.305: RH6.2 RH7.1 78.59,5.08 v83.82,5.08
N$84  (via drill 0.35)
  Top 0.305: v93.98,5.08 93.34,5.08 K7.6
  Bottom 0.305: RH7.2 RH8.1 88.75,5.08 v93.98,5.08
N$85  (via drill 0.35)
  Top 0.305: v104.14,5.08 103.5,5.08 K8.6
  Bottom 0.305: RH8.2 RH9.1 98.91,5.08 v104.14,5.08
N$86  (via drill 0.35)
  Top 0.305: v114.3,5.08 113.66,5.08 K9.6
  Bottom 0.305: RH9.2 RH10.1 109.07,5.08 v114.3,5.08
N$87  (via drill 0.35)
  Top 0.305: v124.46,5.08 123.82,5.08 K10.6
  Bottom 0.305: RH10.2 RH11.1 119.23,5.08 v124.46,5.08
N$88  (via drill 0.35)
  Top 0.305: v27.94,15.24 28.11,15.41 QS1.1
  Bottom 0.305: v27.94,15.24 27.94,15.39 RS1.1
N$89  (via drill 0.35)
  Top 0.508: QS1.3 30.48,11.43 | 30.48,11.43 30.48,10.67 v29.97,10.16 | K1.8 30.49,11.42 30.48,11.43
  Bottom 0.508: DS1.A 29.99,10.14 v29.97,10.16
N$90  (via drill 0.35)
  Top 0.305: QS2.1 38.27,15.41 v38.1,15.24
  Bottom 0.305: v38.1,15.24 39.22,16.36 RS2.1
N$91  (via drill 0.35)
  Top 0.508: QS2.3 40.64,11.43 | 40.64,11.43 40.64,10.67 v40.13,10.16 | K2.8 40.65,11.42 40.64,11.43
  Bottom 0.508: DS2.A 40.15,10.14 v40.13,10.16
N$92  (via drill 0.35)
  Top 0.305: QS3.1 49.68,15.24 v48.26,15.24
  Bottom 0.305: v48.26,15.24 49.38,16.36 RS3.1
N$93  (via drill 0.35)
  Top 0.508: QS3.3 50.8,11.43 | 50.8,11.43 50.8,10.67 v50.29,10.16 | K3.8 50.81,11.42 50.8,11.43
  Bottom 0.508: DS3.A 50.31,10.14 v50.29,10.16
N$94  (via drill 0.35)
  Top 0.305: QS4.1 58.59,15.41 v58.42,15.24
  Bottom 0.305: v58.42,15.24 59.54,16.36 RS4.1
N$95  (via drill 0.35)
  Top 0.508: QS4.3 60.96,11.43 | 60.96,11.43 60.96,10.67 v60.45,10.16 | K4.8 60.97,11.42 60.96,11.43
  Bottom 0.508: DS4.A 60.47,10.14 v60.45,10.16
N$96  (via drill 0.35)
  Top 0.305: QS5.1 70,15.24 v68.58,15.24
  Bottom 0.305: v68.58,15.24 69.7,16.36 RS5.1
N$97  (via drill 0.35)
  Top 0.508: QS5.3 71.12,11.43 | 71.12,11.43 71.12,10.67 v70.61,10.16 | K5.8 71.13,11.42 71.12,11.43
  Bottom 0.508: DS5.A 70.63,10.14 v70.61,10.16
N$98  (via drill 0.35)
  Top 0.305: QS6.1 78.91,15.41 v78.74,15.24
  Bottom 0.305: v78.74,15.24 79.86,16.36 RS6.1
N$99  (via drill 0.35)
  Top 0.508: QS6.3 81.28,11.43 | 81.28,11.43 81.28,10.67 v80.77,10.16 | K6.8 81.29,11.42 81.28,11.43
  Bottom 0.508: DS6.A 80.79,10.14 v80.77,10.16
N$100  (via drill 0.35)
  Top 0.305: QS7.1 90.32,15.24 v88.9,15.24
  Bottom 0.305: v88.9,15.24 88.9,15.39 RS7.1
N$101  (via drill 0.35)
  Top 0.508: QS7.3 91.44,11.43 | 91.44,11.43 91.44,10.67 v90.93,10.16 | K7.8 91.45,11.42 91.44,11.43
  Bottom 0.508: DS7.A 90.95,10.14 v90.93,10.16
N$102  (via drill 0.35)
  Top 0.305: QS8.1 99.23,15.41 v99.06,15.24
  Bottom 0.305: v99.06,15.24 100.18,16.36 RS8.1
N$103  (via drill 0.35)
  Top 0.508: QS8.3 101.6,11.43 | 101.6,11.43 101.6,10.67 v101.09,10.16 | K8.8 101.61,11.42 101.6,11.43
  Bottom 0.508: DS8.A 101.11,10.14 v101.09,10.16
N$104  (via drill 0.35)
  Top 0.305: QS9.1 109.39,15.41 v109.22,15.24
  Bottom 0.305: v109.22,15.24 110.34,16.36 RS9.1
N$105  (via drill 0.35)
  Top 0.508: QS9.3 111.76,11.43 | 111.76,11.43 111.76,10.67 v111.25,10.16 | K9.8 111.77,11.42 111.76,11.43
  Bottom 0.508: DS9.A 111.27,10.14 v111.25,10.16
N$106  (via drill 0.35)
  Top 0.305: QS10.1 119.55,15.41 v119.38,15.24
  Bottom 0.305: v119.38,15.24 120.5,16.36 RS10.1
N$107  (via drill 0.35)
  Top 0.508: QS10.3 121.92,11.43 | 121.92,11.43 121.92,10.67 v121.41,10.16 | K10.8 121.93,11.42 121.92,11.43
  Bottom 0.508: DS10.A 121.43,10.14 v121.41,10.16
N$108  (via drill 0.35)
  Top 0.305: K11.3 124.79,6.02 124.46,6.35 v124.46,21.59
  Bottom 0.305: v124.46,21.59 125.73,22.86 COQ1.1
N$109  (via drill 0.35)
  Top 0.305: K12.3 137.62,6.02 v137.67,5.97 | v149.86,5.97 149.86,13.08 148.59,14.35 v148.59,24.13
  Bottom 0.305: v137.67,5.97 v149.86,5.97 | v148.59,24.13 COQ2.1
N$110  (via drill 0.35)
  Top 0.305: K13.3 145.11,6.02 144.78,6.35 144.78,12.7 146.05,13.97 v146.05,19.05
  Bottom 0.305: v146.05,19.05 149.86,19.05 151.13,20.32 COQ3.2
N$111  (via drill 0.35)
  Top 0.305: QS11.1 129.71,15.41 v129.54,15.24
  Bottom 0.305: v129.54,15.24 130.66,16.36 RS11.1
N$112  (via drill 0.35)
  Top 0.508: QS11.3 132.08,11.43 | 132.08,11.43 132.08,10.67 v131.57,10.16 | K11.8 132.09,11.42 132.08,11.43
  Bottom 0.508: DS11.A 131.59,10.14 v131.57,10.16
N$113  (via drill 0.35)
  Top 0.305: QS12.1 139.87,15.41 v139.7,15.24
  Bottom 0.305: v139.7,15.24 140.82,16.36 RS12.1
N$114  (via drill 0.35)
  Top 0.508: QS12.3 142.24,11.43 | 142.24,11.43 142.24,10.67 v141.73,10.16 | K12.8 142.25,11.42 142.24,11.43
  Bottom 0.508: DS12.A 141.75,10.14 v141.73,10.16
N$115  (via drill 0.35)
  Top 0.305: QS13.1 150.03,15.41 v149.86,15.24
  Bottom 0.305: v149.86,15.24 150.98,16.36 RS13.1
N$116  (via drill 0.35)
  Top 0.508: v151.89,10.16 152.4,10.67 152.4,11.43 | QS13.3 152.4,11.43 | K13.8 152.41,11.42 152.4,11.43
  Bottom 0.508: DS13.A 151.91,10.14 v151.89,10.16
N$117  (via drill 0.35)
  Top 0.305: QS20.1 28.91,34.46 v27.94,35.43
  Bottom 0.305: v27.94,35.43 28.07,35.56 RS20.1
N$118  (via drill 0.35)
  Top 0.508: QS20.3 30.48,30.48 | 30.48,30.48 30.48,29.84 v29.97,29.34 | K20.8 30.49,30.47 30.48,30.48
  Bottom 0.508: v29.97,29.34 29.97,27.96
  Bottom 1.016: 29.97,27.96 DS20.A
N$119
  Bottom 0.305: C211.2 41.78,58.42 35.69,58.42 C210.2 32.51,59.82 31.75,60.58 L1.2
N$120
  Top 0.305: K22.5 49.65,22.87 48.26,24.26 48.26,32.91 47.45,33.72 47.45,39.95 48.39,40.89 48.39,44.07 46.99,45.47 C4.2
  Bottom 0.305: C4.2 45.53,46.95 R44.2 R45.2
N$121
  Bottom 0.305: L2.1 L1.1
N$122
  Bottom 0.305: L2.2 L3.2
N$123
  Bottom 0.305: L4.1 L3.1
N$124
  Top 0.305: K22.4 44.76,23.14 47.8,26.18 47.8,32.72 46.99,33.53 C4.1
  Bottom 0.305: C4.1 45.53,41.95 R44.1
N$125
  Bottom 0.305: D10.1 D11.2
N$126  (via drill 0.35)
  Top 0.305: K23.4 57.96,25.91 57.96,30.82 57.15,31.63 57.15,32.64 55.88,33.91 v55.88,40.13
  Bottom 0.305: v55.88,40.13 51.82,40.13 50.8,41.15 R46.1
N$127  (via drill 0.35)
  Top 0.305: QS22.1 48.43,34.46 v48.26,34.29
  Bottom 0.305: v48.26,34.29 49.38,35.41 RS22.1
N$128  (via drill 0.35)
  Top 0.508: v50.29,29.34 50.8,29.84 50.8,30.48 | QS22.3 50.8,30.48 | K22.8 50.81,30.47 50.8,30.48
  Bottom 0.508: DS22.A 50.31,29.32 v50.29,29.34
N$129  (via drill 0.35)
  Top 0.305: QS23.1 58.59,34.46 v58.42,34.29
  Bottom 0.305: v58.42,34.29 59.54,35.41 RS23.1
N$130  (via drill 0.35)
  Top 0.508: v60.45,29.34 60.96,29.84 60.96,30.48 | QS23.3 60.96,30.48 | K23.8 60.97,30.47 60.96,30.48
  Bottom 0.508: DS23.A 60.47,29.32 v60.45,29.34
N$131  (via drill 0.35)
  Top 0.305: QS24.1 68.75,34.46 v68.58,34.29
  Bottom 0.305: v68.58,34.29 69.7,35.41 RS24.1
N$132  (via drill 0.35)
  Top 0.508: v70.61,29.26 71.12,29.77 71.12,30.48 | QS24.3 71.12,30.48 | K24.8 71.13,30.47 71.12,30.48
  Bottom 0.61: DS24.A 70.63,29.24 v70.61,29.26
N$133  (via drill 0.35)
  Top 0.305: v66.29,40.13 66.29,32.65 68.12,30.82 68.12,25.91 K24.4
  Bottom 0.305: v66.29,40.13 62.87,40.13 62.23,40.77 R48.1
N$134  (via drill 0.35)
  Top 0.305: K23.5 59.3,22.87 58.42,23.75 58.42,31.01 57.66,31.77 v57.66,46.86
  Bottom 0.305: R46.2 51.88,46.95 C3.2 57.57,46.95 v57.66,46.86 58.7,46.86 R47.2
N$135
  Bottom 0.305: D8.1 D7.2
N$136
  Bottom 0.305: D7.1 D6.2
N$137
  Top 0.305: K24.5 69.46,22.87 68.58,23.75 68.58,31.24 67.18,32.64 67.18,44.54 C5.2
  Bottom 0.305: R48.2 63.31,46.95 C5.2 66.23,46.95 R49.2 67.59,45.87 C222.1
N$138  (via drill 0.35)
  Top 0.305: C46.+ 177.65,70.97 v177.8,71.12
  Bottom 0.305: v177.8,71.12 R104.2
N$139  (via drill 0.35)
  Top 0.305: v140.97,52.32 142.14,52.32 C47.-
  Bottom 0.305: R111.2 141.07,52.22 v140.97,52.32
N$140  (via drill 0.35)
  Top 0.305: QS15.1 110.64,34.29 v109.22,34.29
  Bottom 0.305: v109.22,34.29 110.34,35.41 RS15.1
N$141  (via drill 0.35)
  Top 0.508: v111.25,29.34 111.76,29.84 111.76,30.48 | QS15.3 111.76,30.48 | K15.8 111.76,30.48
  Bottom 0.508: DS15.A 111.27,29.32 v111.25,29.34
N$142  (via drill 0.35)
  Top 0.305: QS16.1 119.55,34.46 v119.38,34.29
  Bottom 0.305: v119.38,34.29 120.5,35.41 RS16.1
N$143  (via drill 0.35)
  Top 0.508: v121.41,29.34 121.92,29.84 121.92,30.48 | QS16.3 121.92,30.48 | K16.8 121.93,30.47 121.92,30.48
  Bottom 0.508: DS16.A 121.43,29.32 v121.41,29.34
N$144  (via drill 0.35)
  Top 0.305: QS17.1 78.91,34.46 v78.74,34.29
  Bottom 0.305: v78.74,34.29 79.86,35.41 RS17.1
N$145  (via drill 0.35)
  Top 0.508: v80.77,29.34 81.28,29.84 81.28,30.48 | QS17.3 81.28,30.48 | K17.8 81.29,30.47 81.28,30.48
  Bottom 0.508: v80.77,29.34 80.77,27.96
  Bottom 1.016: 80.77,27.96 DS17.A
N$146  (via drill 0.35)
  Top 0.305: QS18.1 89.07,34.46 v88.9,34.29
  Bottom 0.305: v88.9,34.29 90.02,35.41 RS18.1
N$147  (via drill 0.35)
  Top 0.508: QS18.3 91.44,30.48 | 91.44,30.48 91.44,29.84 v90.93,29.34 | K18.8 91.44,30.48
  Bottom 0.508: v90.93,29.34 90.95,29.32 DS18.A
N$148  (via drill 0.35)
  Top 0.305: QS21.1 39.52,34.29 v38.1,34.29
  Bottom 0.305: v38.1,34.29 39.22,35.41 RS21.1
N$149  (via drill 0.35)
  Top 0.508: v40.13,29.34 40.64,29.84 40.64,30.48 | QS21.3 40.64,30.48 | K21.8 40.65,30.47 40.64,30.48
  Bottom 0.508: v40.13,29.34 40.13,27.96
  Bottom 1.016: 40.13,27.96 DS21.A
N$150  (via drill 0.35)
  Top 0.305: IC1.9 v21.08,24.77 | IC2.14 135.64,31.11 136.14,30.61 v136.14,25.65
  Bottom 0.305: v21.08,24.77 21.46,24.38 75.18,24.38 76.45,25.65 130.93,25.65 130.94,25.65 v136.14,25.65
N$151  (via drill 0.35)
  Top 0.305: v135.89,23.5 135.89,24.38 135.51,24.77 IC2.9 | IC3.14 22.23,12.06 22.86,12.7 22.86,18.9 v22.18,19.59
  Bottom 0.305: v22.18,19.59 22.35,19.76 83.21,19.76 83.56,19.41 84.44,19.41 85.24,20.22 96.42,20.22 96.77,19.87 97.85,19.87 98.65,20.68 103.53,20.68 103.88,20.33 104.4,20.33 105.21,21.13 122.1,21.13 124.46,23.5 v135.89,23.5
N$152  (via drill 0.35)
  Top 0.305: v134.62,5.08 133.68,6.02 K11.6
  Bottom 0.305: v134.62,5.08 135.89,3.81 157.48,3.81 CPR1.1
N$153  (via drill 0.35)
  Top 0.305: v144.78,5.08 143.84,6.02 K12.6
  Bottom 0.305: v144.78,5.08 156.21,5.08 157.48,6.35 CPR2.1
N$154  (via drill 0.35)
  Top 0.305: CPR3.2 v171.45,7.62 | v154.94,7.62 154.94,7.6 K13.6
  Bottom 0.305: v171.45,7.62 167.02,7.62 166.56,8.08 163.64,8.08 163.18,7.62 v154.94,7.62
N$155  (via drill 0.35)
  Top 0.305: v158.75,16.51 157.48,17.78 COQ4.1
  Bottom 0.305: ROQ4.2 v158.75,16.51
N$156
  Bottom 0.305: RPR4.2 176.68,6.2 177.8,5.08 CPR4.1
N$157  (via drill 0.35)
  Top 0.305: IC22.3 v146.05,49.53
  Bottom 0.305: v146.05,49.53 145.9,49.38 R111.1
N$158  (via drill 0.35)
  Top 0.305: IC22.5 149.48,46.99 149.86,46.61 v149.86,45.72
  Bottom 0.305: v149.86,45.72 R114.1
N$159  (via drill 0.35)
  Top 0.305: IC22.2 v146.05,50.8
  Bottom 0.305: R118.1 157.33,50.8 v146.05,50.8
N$160  (via drill 0.35)
  Top 0.305: v159.38,48.13 159.38,43.66 C49.-
  Bottom 0.305: R118.2 159.36,48.11 v159.38,48.13
N$161  (via drill 0.35)
  Top 0.305: IC22.1 148.34,52.07 148.72,51.69 148.72,48.64 148.34,48.26 IC22.4 145.03,48.26 144.78,48.01 v144.78,45.59
  Bottom 0.305: R110.1 R109.2 v144.78,45.59
N$162  (via drill 0.35)
  Top 0.305: IC22.8 v153.67,44.45
  Bottom 0.305: v153.67,44.45 156.06,44.45 R112.1
N$163  (via drill 0.35)
  Top 0.305: v148.59,45.72 IC22.6
  Bottom 0.305: R115.2 148.44,45.72 v148.59,45.72
N$164  (via drill 0.35)
  Top 0.305: IC22.12 v154.94,49.53 | v162.56,50.8 162.41,50.95 C48.+
  Bottom 0.305: v154.94,49.53 161.29,49.53 v162.56,50.8 R116.1
N$165  (via drill 0.35)
  Top 0.305: C48.- v161.29,46.61 | IC23.2 170.56,45.09 170.81,45.34 v170.81,47.37 v170.82,47.37 170.03,48.16 R117.1
  Bottom 0.305: v161.29,46.61 166.37,46.61 167.13,47.37 v170.82,47.37
N$166  (via drill 0.35)
  Top 0.305: IC22.10 v154.94,46.99 156.46,46.99 157.48,48.01 157.48,55.73 R99.2
  Bottom 0.305: v154.94,46.99 157.48,46.99 157.49,47 158.75,47 | R124.1 160.25,48.11 159.15,47 158.75,47 | R113.1 158.75,47
N$167  (via drill 0.35)
  Top 0.305: v166.88,56.52 IC24.2 170.81,56.52 | v171.45,49.53 171.45,55.88 170.81,56.52 | 170.81,56.52 170.81,61.59 C51.1
  Bottom 0.305: v166.88,56.52 166.09,57.3 R122.2 | R121.2 v171.45,49.53
N$168  (via drill 0.35)
  Top 0.305: v178.05,49.53 178.05,45.04 D5.1
  Bottom 0.305: R121.1 v178.05,49.53
N$169  (via drill 0.35)
  Top 0.305: D4.2 182.29,51.23 v181.99,50.93
  Bottom 0.305: R119.1 181.97,50.95 v181.99,50.93 184.12,50.93 R120.2
N$170  (via drill 0.35)
  Top 0.305: D5.2 182.88,43.61 182.88,47.12 v181.86,48.13 | C50.+ v179.07,46.76
  Bottom 0.305: v181.86,48.13 180.37,48.13 R119.2 179.43,48.11 179.07,47.75 v179.07,46.76
R01  (via drill 0.35)
  Top 0.305: v9.53,13.97 9.53,7.49 10.03,6.99 IC3.7
  Bottom 0.305: v9.53,13.97 30.99,13.97 31.9,14.88 RS1.2
R02  (via drill 0.35)
  Top 0.305: v10.16,11.81 10.16,8.64 10.54,8.26 IC3.6
  Bottom 0.305: v10.16,11.81 11.86,13.51 41.45,13.51 42.06,14.12 RS2.2
R03  (via drill 0.35)
  Top 0.305: v10.92,11.43 10.92,9.78 11.18,9.53 IC3.5
  Bottom 0.305: v10.92,11.43 12.55,13.06 51.16,13.06 52.22,14.12 RS3.2
R04  (via drill 0.35)
  Top 0.305: v11.55,10.79 IC3.4
  Bottom 0.305: v11.55,10.79 13.36,12.6 60.86,12.6 62.38,14.12 RS4.2
R05  (via drill 0.35)
  Top 0.305: v10.5,18.67 10.5,12.36 10.79,12.06 IC3.3
  Bottom 0.305: v10.5,18.67 10.8,18.67 11,18.47 12.39,18.47 12.77,18.85 19.51,18.85 21.24,17.11 23.12,17.11 23.94,17.93 72.24,17.93 72.54,17.63 RS5.2
R06  (via drill 0.35)
  Top 0.305: IC3.2 11.56,13.34 11.13,13.76 v11.13,19.24
  Bottom 0.305: v11.13,19.24 11.37,19.24 11.68,18.93 12.2,18.93 12.58,19.3 19.9,19.3 21.64,17.57 22.93,17.57 23.75,18.39 82.45,18.39 82.7,18.14 RS6.2
R07  (via drill 0.35)
  Top 0.305: v11.94,19.56 11.94,14.99 12.32,14.61 IC3.1
  Bottom 0.305: v11.94,19.56 12.14,19.76 20.09,19.76 21.83,18.03 22.74,18.03 23.56,18.85 82.83,18.85 83.21,18.47 92.28,18.47 92.86,17.88 RS7.2
R08  (via drill 0.35)
  Top 0.305: IC3.15 21.97,13.34 22.4,13.77 22.4,18.35 v22.09,18.66
  Bottom 0.305: v22.09,18.66 v22.1,18.67 22.73,18.67 23.37,19.3 83.02,19.3 83.4,18.92 101.6,18.92 101.73,18.92 103.02,17.63 RS8.2
R09  (via drill 0.35)
  Top 0.305: v125.73,17.91 125.73,25.65 126.11,26.04 IC2.7
  Bottom 0.305: v125.73,17.91 114.56,17.91 113.18,16.53 RS9.2
R10  (via drill 0.35)
  Top 0.305: v125.09,16.51 125.09,27.05 125.35,27.3 IC2.6
  Bottom 0.305: v125.09,16.51 RS10.2
R11  (via drill 0.35)
  Top 0.305: v129.79,18.41 129.79,27.94 129.16,28.57 IC2.5
  Bottom 0.305: RS11.2 133.5,17.63 132.72,18.41 v129.79,18.41
R12  (via drill 0.35)
  Top 0.305: IC2.4 129.67,29.84 130.43,29.08 v130.43,19.05
  Bottom 0.305: RS12.2 143.66,17.88 142.5,19.05 v130.43,19.05
R13  (via drill 0.35)
  Top 0.305: v153.67,17.78 153.67,27.69 v153.16,28.19 | v129.54,31.11 IC2.3
  Bottom 0.305: v129.54,31.11 130.18,30.48 135.89,30.48 137.16,29.21 142.88,29.21 143.89,28.19 151.13,28.19 v153.16,28.19 | v153.67,17.78 153.82,17.63 RS13.2
R15  (via drill 0.35)
  Top 0.305: IC2.1 v125.73,33.66
  Bottom 0.305: v125.73,33.66 116.84,33.66 114.94,35.56 RS15.2
R16  (via drill 0.35)
  Top 0.305: v135.89,36.07 135.89,33.02 135.25,32.38 IC2.15
  Bottom 0.305: v135.89,36.07 135.64,36.32 124.1,36.32 RS16.2
R17  (via drill 0.35)
  Top 0.305: v83.82,35.56 v83.82,20.04 | v11.23,20.04 11.23,25.2 12.06,26.04 IC1.7
  Bottom 0.305: v83.82,20.04 83.64,20.22 11.4,20.22 v11.23,20.04 | v83.82,35.56 RS17.2
R18  (via drill 0.35)
  Top 0.305: IC1.6 10.92,27.3 10.54,26.92 v10.54,20.5 | v97.03,20.5 97.03,28.19 96.52,28.7 94.61,28.7 93.98,29.34 93.98,35.31 v94.11,35.43
  Bottom 0.305: v10.54,20.5 10.72,20.68 96.85,20.68 v97.03,20.5 | v94.11,35.43 93.98,35.56 RS18.2
R19  (via drill 0.35)
  Top 0.305: v104.14,34.29 v104.14,20.96 | v9.91,21.08 9.91,28.07 10.41,28.57 IC1.5
  Bottom 0.305: v104.14,20.96 103.97,21.13 9.96,21.13 v9.91,21.08 | v104.14,34.29 104.14,34.44 RS19.2
R20  (via drill 0.35)
  Top 0.305: v15.88,33.27 15.88,30.23 15.49,29.84 IC1.4
  Bottom 0.305: v15.88,33.27 16.05,33.09 20.51,33.09 21.59,34.18 23.38,34.18 23.73,33.83 31.54,33.83 31.9,34.19 RS20.2
R21  (via drill 0.35)
  Top 0.305: IC1.3 11.56,31.11 11.05,31.62 v11.05,35.56 | v22.86,35.56 22.86,33.8 v23.11,33.55
  Bottom 0.305: v11.05,35.56 11.69,36.2 22.23,36.2 v22.86,35.56 | v23.11,33.55 23.29,33.37 41.76,33.37 42.06,33.68 RS21.2
R22  (via drill 0.35)
  Top 0.305: IC1.2 13.69,32.64 v15.11,32.64
  Bottom 0.305: v15.11,32.64 20.7,32.64 21.33,33.27 22.5,33.27 22.85,32.92 51.59,32.92 52.22,33.55 RS22.2
R23  (via drill 0.35)
  Top 0.305: IC1.1 12.06,33.66 11.68,34.04 v11.68,36.96
  Bottom 0.305: v11.68,36.96 12.06,37.34 61.72,37.34 62.38,36.68 RS23.2
R24  (via drill 0.35)
  Top 0.305: IC1.15 21.34,32.38 v21.59,32.64 | v74.17,32.63 v74.17,35.56
  Bottom 0.305: v21.59,32.64 v21.59,32.63 22.49,32.63 22.66,32.46 73.99,32.46 v74.17,32.63 | v74.17,35.56 RS24.2
SDIN  (via drill 0.35)
  Top 0.305: v17.65,30.62 18.14,31.11 IC1.14 | v5.08,29.21 5.08,31.75 CON2.8
  Bottom 0.305: v17.65,30.62 10.19,30.62 8.91,29.35 5.22,29.35 v5.08,29.21
SHCP  (via drill 0.35)
  Top 0.305: v22.23,32 22.23,30.86 22.05,30.68 22.05,27.3 | IC1.11 22.05,27.3 | IC2.11 v135.25,27.3 | v136.91,32.26 v136.91,27.3 | IC3.11 22.73,8.26 23.11,8.64 23.11,12.19 23.32,12.39 23.32,19.35 22.05,20.62 22.05,27.3
  Bottom 0.305: CON2.7 8.76,33.02 9.78,32 v22.22,32 v22.23,32 128.89,32 129.09,32.2 136.85,32.2 v136.91,32.26 | v135.25,27.3 v136.91,27.3
STCP  (via drill 0.35)
  Top 0.305: IC2.12 132.59,28.57 132.08,29.08 v132.08,31.37 | IC1.12 21.46,28.57 21.59,28.7 v21.59,31.37 | IC3.12 v21.21,9.53 | v8.89,9.4 v8.89,30.61
  Bottom 0.305: v132.08,31.37 130.18,31.37 129.8,31.75 129.28,31.75 128.9,31.37 v21.59,31.37 9.65,31.37 v8.89,30.61 8.76,30.48 CON2.5 | v21.21,9.53 9.02,9.53 v8.89,9.4

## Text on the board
tDocu: C(OQ) | C(PR) | R(G) | AMPL. | R(H) | FREQ. | POWER / SUPPLY | QREF | FCONT | ACONT | IREF | Mica | Mica | Mica | MPET | MPET | THD-Analyzer B Cordell / PCB2 v0.21 by Emile / 05-2022 | DIST. | Mica | MPET | GND | PRODUCT / AMPLIFIER / AND / LEVEL SET | INPUT / CIRCUIT | AGC | Mica | Mica | D S G | D S G | 10 V | 30 V | 100 V | VOLTAGE CONTROLLED / BANDPASS FILTER | Mica | MPET | MPET | MPET | RELAYS AND DIGITAL LOGIC | ANALOG / INTERFACE | MPET | MPET | MPET | Mica
bDocu: THD-Analyzer B Cordell / PCB2 v0.21 by Emile / Bottom-Layer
